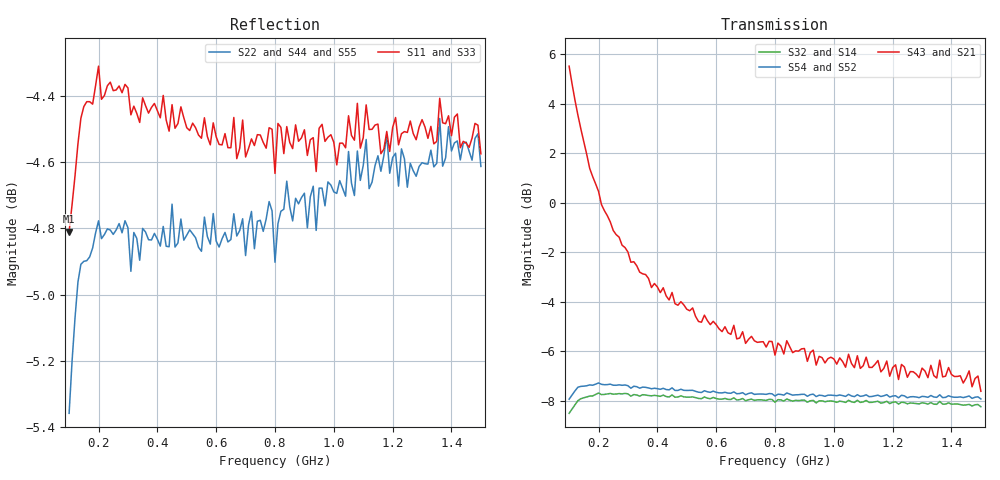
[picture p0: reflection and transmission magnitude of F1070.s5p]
!  POLYFET RF DEVICES
!  S PARAMETERS FOR
!  F1070 (Each Side)
!  VDS=28, IDQ=800mA
! Date: Nov 11, 1991
! Bias (V mA) : V1=3.5470000  I1=0.0070885  V2=27.990760  I2=768.13320
!AWR Design Environment (2053) Wed Feb 04 14:45:42 2004
!freq-unit  param-type  data-format  keyword  impedance-ohms
# MHz  S  MA  R  50
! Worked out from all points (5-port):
!   141 points, 100 MHz to 1.5 GHz, reference 50 ohm
!   strongest paths, dB at 100 MHz, 450 MHz, 800 MHz, 1.15 GHz, 1.5 GHz:
!     S43: 5.5, -3.6, -6.2, -6.4, -7.6
!     S21: 5.5, -3.6, -6.2, -6.4, -7.6
!     S54: -7.9, -7.5, -7.8, -7.8, -7.9
!     S52: -7.9, -7.5, -7.8, -7.8, -7.9
!     S32: -8.5, -7.8, -8.1, -8.0, -8.2
!     S14: -8.5, -7.8, -8.1, -8.0, -8.2
!   lowest |S11| = -4.8 dB at 100 MHz (marker M1), VSWR 3.70, Z = 15.4 - j17.9 ohm
!   |S11| at or under -10 dB: nowhere
